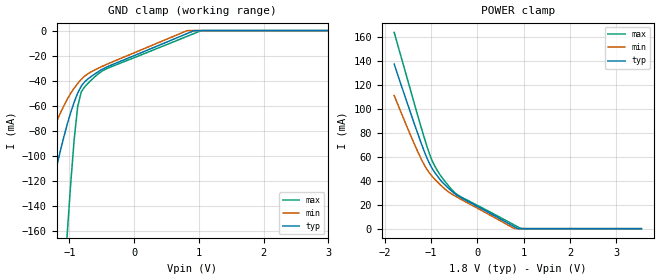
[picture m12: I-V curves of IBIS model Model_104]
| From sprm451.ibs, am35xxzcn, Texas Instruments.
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| Model based on original model for BSSTL18TCSCGPBFZ_7LM
|   Sub model FULL_TERM_SSTL_1P8
[model]   Model_104
|[Description]  1.8V-INPUT-FULL_SSTL-X-+-10%V
|[Input Load]   FULL_SSTL
|[Output Drive]
|Voltage   1.8V
|Mode   INPUT
Model_type   Input
Polarity   Non-Inverting
Vinl =  0.8
Vinh =  1
C_comp   3.009089p   2.23501p   3.950269p
[Model Spec]
Vinl   0.8   0.71   0.89
Vinh   1   0.91   1.09
[Temperature Range]   25   125   -40
[Voltage Range]   1.8   1.62   1.98
[POWER_clamp]
-1.8V     137.1mA    110.9mA    163.5mA
-1.309V   81.24mA    65.7mA     96.68mA
-1.145V   63.98mA    52.82mA    75.18mA
-1.036V   54.18mA    46.26mA    62.21mA
-927.3mV  47.05mA    41.38mA    52.44mA
-818.2mV  41.41mA    37.14mA    45.43mA
-600mV    32.76mA    29.93mA    34.49mA
-436.4mV  27.7mA     26.15mA    28.33mA
763.6mV   2.335mA    781.1uA    3.756mA
872.7mV   0A         0A         1.482mA
981.8mV   0A         0A         0A
3.545V    0A         0A         0A
[GND_clamp]
-1.8V     -248.2mA   -152.9mA   -828.2mA
-1.418V   -158.5mA   -100.4mA   -490.9mA
-1.2V     -108.8mA   -72.76mA   -299.5mA
-1.036V   -75.1mA    -54.98mA   -163.6mA
-927.3mV  -57.07mA   -45.94mA   -86.82mA
-872.7mV  -49.87mA   -42.18mA   -60.55mA
-818.2mV  -44.34mA   -38.92mA   -48.93mA
-763.6mV  -40.8mA    -36.25mA   -44.82mA
-490.9mV  -30.82mA   -28.47mA   -32.17mA
818.2mV   -2.352mA   -40.93uA   -4.565mA
1.036V    0A         0A         0A
3.545V    0A         0A         0A
